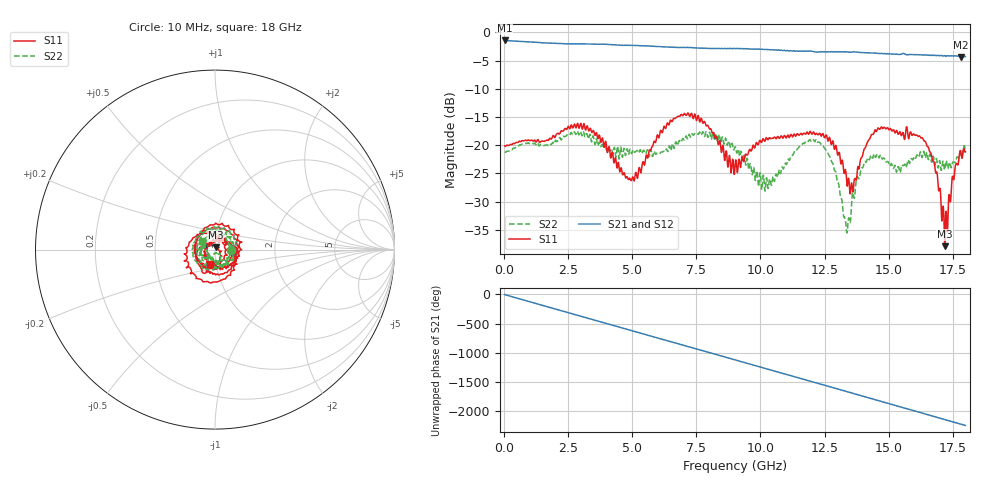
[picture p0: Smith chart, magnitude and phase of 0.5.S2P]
!Agilent Technologies,E5071C,MY46316741,A.11.02
!Date: Fri May 06 15:18:32 2022
!Data & Calibration Information:
!Freq	S11:SOLT2(ON)	S21:SOLT2(ON)	S12:SOLT2(ON)	S22:SOLT2(ON)
!PortZ  Port1:50+j0  Port2:50+j0
!Above PortZ is port z conversion or system Z0 setting when saving the data.
!When reading, reference impedance value at option line is always used.
# Hz S dB R 50
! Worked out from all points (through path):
!   1800 points, 10 MHz to 18 GHz, reference 50 ohm
!   highest |S21| = -1.44 dB at 10 MHz (marker M1); lowest = -4.4 dB at 17.83 GHz (marker M2)
!   group delay of S21, straight-line fit = 347 ps
!   lowest |S11| = -37.9 dB at 17.19 GHz (marker M3), VSWR 1.03, Z = 50.5 + j1.19 ohm
!   |S11| at or under -10 dB: start of sweep to end of sweep
!   |S22| runs from -35.5 to -17.5 dB; largest |S21 - S12| = 0.051
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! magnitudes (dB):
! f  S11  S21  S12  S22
! 10 MHz  -20.1  -1.4  -1.5  -21.2
! 3.01 GHz  -16.5  -2.0  -2.1  -18.1
! 3.77 GHz  -19.5  -2.1  -2.1  -20.3
! 4.9 GHz  -25.9  -2.3  -2.3  -20.8
! 6.01 GHz  -18.6  -2.5  -2.5  -21.3
! 7.37 GHz  -15.3  -2.7  -2.8  -18.2
! 9.01 GHz  -23.5  -2.9  -2.9  -20.3
! 10.24 GHz  -18.7  -3.1  -3.1  -25.8
! 12.01 GHz  -18.0  -3.3  -3.4  -19.1
! 12.76 GHz  -19.9  -3.4  -3.5  -22.7
! 13.41 GHz  -26.5  -3.5  -3.5  -34.2
! 13.67 GHz  -26.0  -3.5  -3.5  -29.3
! 14.12 GHz  -20.1  -3.6  -3.7  -23.0
! 15.01 GHz  -17.3  -3.8  -3.8  -23.1
! 15.39 GHz  -18.0  -3.9  -4.0  -23.8
! 16.4 GHz  -19.3  -4.0  -4.1  -21.5
! 16.83 GHz  -24.6  -4.1  -4.1  -23.1
! 17.19 GHz  -37.9  -4.1  -4.2  -24.4
! 17.25 GHz  -31.7  -4.2  -4.2  -22.7
! 17.55 GHz  -26.1  -4.2  -4.3  -23.0
! 17.83 GHz  -21.4  -4.4  -4.4  -20.9
! 18 GHz  -21.2  -4.3  -4.4  -21.1
